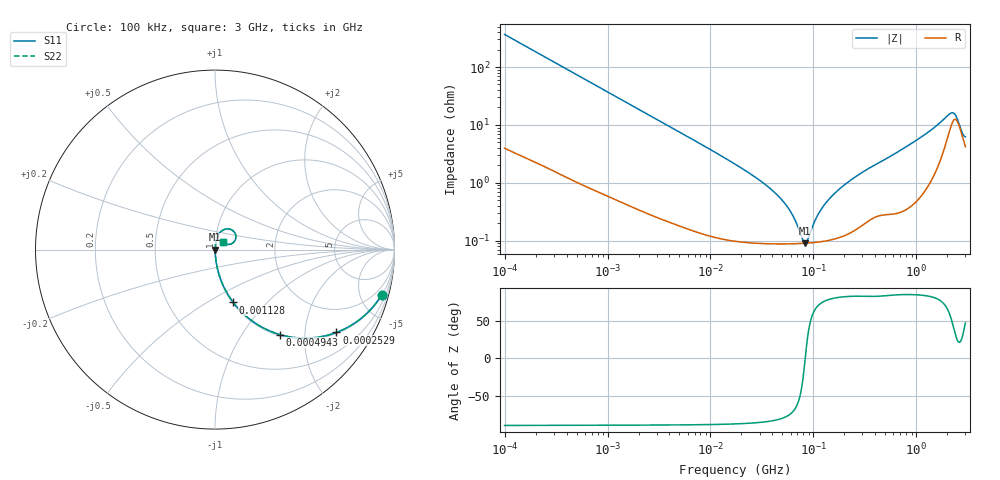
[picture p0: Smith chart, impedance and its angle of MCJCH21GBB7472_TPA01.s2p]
! MCJCH21GBB7472_TPA01  S-PARAMETER MODEL  ( Standard Model )
! Model Generated by TAIYO YUDEN Corporation (http://www.ty-top.com)
! Version 1.0
! TAIYO YUDEN Control No. 220601
! Copyright(c) 2015 TAIYO YUDEN CO.,LTD. All Rights Reserved.
! Product Description (link to TY-COMPAS)
! https://ds.yuden.co.jp/TYCOMPAS/or/detail?pn=MCJCH21GBB7472KTPA01&u=M
! Products Name : Multilayer Ceramic Capacitors
! Characteristics :
!  Capacitance : 4700 [pF] , Rated Voltage : 100 [V] , TCC : X7R
!  Case Size : 2.0 x 1.25 / 0.079 x 0.049 [mm/inch] , Thickness : 1.25 / 0.049 [mm/inch]
!  (Conditions: Temperature = 25 [degC] , DC Bias Voltage = 0 [V])
! External Node Assignments :
!  1  o---| |---o  2
! GND o---------o GND
! Frequency Range : 100kHz  -  3GHz  [ 401 STEP ]
# MHZ S RI R 50
! Freq[MHz].  S11 Real  S11 Imag  S21 Real  S21 Imag  S12 Real  S12 Imag  S22 Real  S22 Imag
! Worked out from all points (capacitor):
!   401 points, 100 kHz to 3 GHz, reference 50 ohm
!   read as one part in series: C = 4.36 nF near 105.3 kHz
!   lowest |Z| = 90.3 mohm at 83.43 MHz (marker M1)
!   series resonance near 83.33 MHz, so ESL is about 840 pH
!   S11 on the Smith chart (normalised r, x): 100 kHz: 1.08, -7.29; 252.9 kHz: 1.04, -2.90; 494.3 kHz: 1.02, -1.49; 1.128 MHz: 1.01, -0.66; 3 GHz: 1.08, +0.09
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0.1  0.9277 -0.2536  0.0723 0.2536  0.0723 0.2536  0.9277 -0.2536
0.252895  0.6761 -0.4616  0.3239 0.4616  0.3239 0.4616  0.6761 -0.4616
0.494258  0.3599 -0.4731  0.6401 0.4731  0.6401 0.4731  0.3599 -0.4731
0.562235  0.3042 -0.4531  0.6958 0.4531  0.6958 0.4531  0.3042 -0.4531
1.127518  0.1019 -0.2945  0.8981 0.2945  0.8981 0.2945  0.1019 -0.2945
3.161081  0.0162 -0.1164  0.9838 0.1164  0.9838 0.1164  0.0162 -0.1164
17.7727  0.00139 -0.0204  0.9986 0.0204  0.9986 0.0204  0.00139 -0.0204
32.98988  0.000983 -0.00972  0.999 0.00972  0.999 0.00972  0.000983 -0.00972
48.55934  0.000905 -0.00517  0.9991 0.00517  0.9991 0.00517  0.000905 -0.00517
61.23616  0.00089 -0.00286  0.9991 0.00286  0.9991 0.00286  0.00089 -0.00286
79.23846  0.000898 -0.00046  0.9991 0.00046  0.9991 0.00046  0.000898 -0.00046
83.42988  0.000903 1.13e-05  0.9991 -1.13e-05  0.9991 -1.13e-05  0.000903 1.13e-05
87.84301  0.000908 0.000482  0.9991 -0.000482  0.9991 -0.000482  0.000908 0.000482
97.38194  0.000924 0.00143  0.9991 -0.00143  0.9991 -0.00143  0.000924 0.00143
122.8043  0.000981 0.00364  0.999 -0.00364  0.999 -0.00364  0.000981 0.00364
167.3121  0.00114 0.00691  0.9989 -0.00691  0.9989 -0.00691  0.00114 0.00691
273.0175  0.00183 0.0135  0.9982 -0.0135  0.9982 -0.0135  0.00183 0.0135
547.5153  0.00359 0.0277  0.9964 -0.0277  0.9964 -0.0277  0.00359 0.0277
1457.883  0.0195 0.0832  0.9805 -0.0832  0.9805 -0.0832  0.0195 0.0832
2145.926  0.0942 0.1095  0.9058 -0.1095  0.9058 -0.1095  0.0942 0.1095
2378.954  0.1166 0.0665  0.8834 -0.0665  0.8834 -0.0665  0.1166 0.0665
3000  0.0422 0.0421  0.9578 -0.0421  0.9578 -0.0421  0.0422 0.0421
